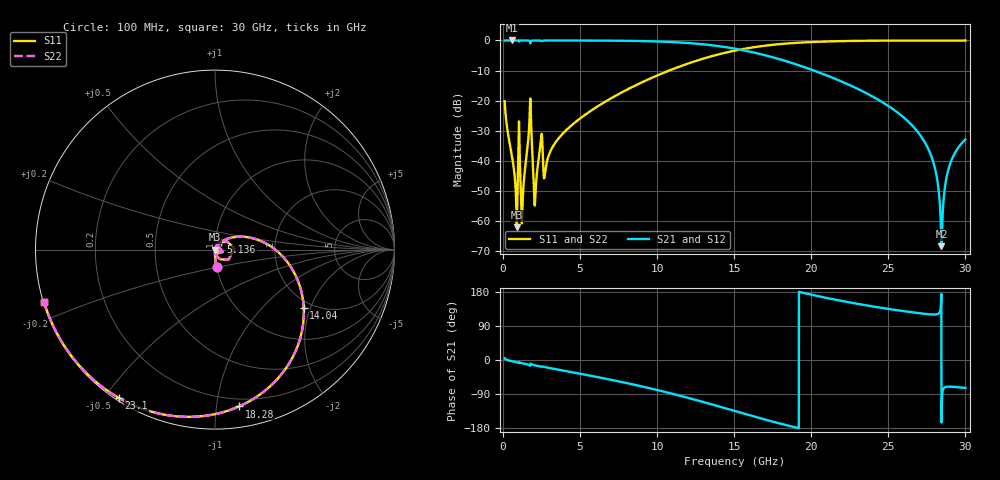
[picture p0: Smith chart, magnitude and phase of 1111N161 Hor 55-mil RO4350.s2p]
# GHz S MA R 50
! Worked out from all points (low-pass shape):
!   3201 points, 100 MHz to 30 GHz, reference 50 ohm
!   highest |S21| = 0.00 dB at 576.5 MHz (marker M1); lowest = -68.4 dB at 28.45 GHz (marker M2)
!   |S21| within 3 dB of the highest: start of sweep to 15.33 GHz
!   lowest |S11| = -62.2 dB at 894.2 MHz (marker M3), VSWR 1.00, Z = 50.1 - j0.00561 ohm
!   |S11| at or under -10 dB: start of sweep to 10.78 GHz
!   |S22| runs from -62.2 to 0.0 dB; largest |S21 - S12| = 0
!   S11 on the Smith chart (normalised r, x): 100 MHz: 1.00, -0.20; 5.136 GHz: 1.07, +0.09; 14.04 GHz: 1.80, -1.80; 18.28 GHz: 0.14, -1.16; 23.1 GHz: 0.01, -0.54; 30 GHz: 0.00, -0.15
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0.1  0.09749 -84.9  0.995 4.9  0.995 4.9  0.09749 -84.9
0.5765313  0.01186 -91.2  0.9994 -3.2  0.9994 -3.2  0.01186 -91.2
0.8942187  0.0007792 -4.1  0.9991 -6.1  0.9991 -6.1  0.0007792 -4.1
1.296  0.002893 64.0  0.999 -9.0  0.999 -9.0  0.002893 64.0
1.725812  0.05729 51.3  0.9751 -14.7  0.9751 -14.7  0.05729 51.3
2.099563  0.002741 38.6  0.9981 -14.4  0.9981 -14.4  0.002741 38.6
2.426594  0.01894 52.4  0.993 -17.4  0.993 -17.4  0.01894 52.4
2.753625  0.007131 51.3  0.9972 -19.0  0.9972 -19.0  0.007131 51.3
5.089563  0.05251 51.8  0.9969 -36.9  0.9969 -36.9  0.05251 51.8
5.136281  0.05359 51.5  0.9968 -37.3  0.9968 -37.3  0.05359 51.5
10.06978  0.266 9.7  0.9607 -79.8  0.9607 -79.8  0.266 9.7
14.04087  0.5916 -33.3  0.8009 -123.0  0.8009 -123.0  0.5916 -33.3
15.05  0.6781 -45.1  0.729 -134.8  0.729 -134.8  0.6781 -45.1
18.28294  0.8839 -81.3  0.4588 -170.9  0.4588 -170.9  0.8839 -81.3
20.03956  0.9417 -98.3  0.325 172.1  0.325 172.1  0.9417 -98.3
23.10431  0.9848 -122.9  0.1525 147.5  0.1525 147.5  0.9848 -122.9
25.01978  0.9934 -135.8  0.08071 134.8  0.08071 134.8  0.9934 -135.8
27.56128  0.9966 -150.6  0.01633 121.0  0.01633 121.0  0.9966 -150.6
28.08453  0.9967 -153.4  0.006425 120.2  0.006425 120.2  0.9967 -153.4
28.44894  0.9968 -155.3  0.0003789 -164.9  0.0003789 -164.9  0.9968 -155.3
28.97219  0.9967 -158.0  0.008323 -70.3  0.008323 -70.3  0.9967 -158.0
30  0.9965 -163.1  0.0225 -73.7  0.0225 -73.7  0.9965 -163.1
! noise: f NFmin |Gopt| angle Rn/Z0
0.1  0.0006576  0.7316  0.958  0.0004884
3.417  0.008861  0.4407  22.6  0.002542
6.743  0.01431  0.3695  41.26  0.003229
10.06  0.02157  0.3937  56.79  0.004663
13.39  0.03228  0.4715  71.5  0.00727
16.7  0.05095  0.5957  88.07  0.01268
20.03  0.09051  0.742  107.2  0.02577
23.35  0.1982  0.8722  127.1  0.0675
26.67  0.7801  0.9653  146  0.439
30  1.252  0.9775  163  0.2825
